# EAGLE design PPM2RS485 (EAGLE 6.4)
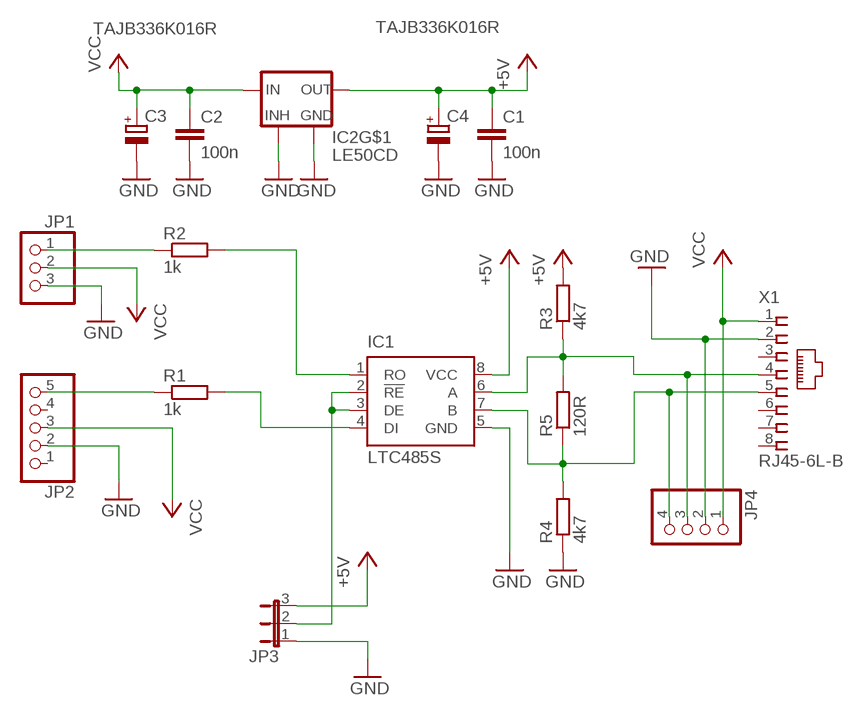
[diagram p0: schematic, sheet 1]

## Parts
C1  100n  C-EU_KOLIN  [M0805]
C2  100n  C-EU_KOLIN  [M0805]
C3  TAJB336K016R  CPOL-EUSMCB  [SMC_B]
C4  TAJB336K016R  CPOL-EUSMCB  [SMC_B]
IC1  LTC485S  [SOIC8]
IC2  LE50CD  LE33CD  [SO8]
JP1  PINHD-1X3  [1X03]
JP2  PINHD-1X5  [1X05]
JP3  JP2E  [JP2]
JP4  PINHD-1X4  [1X04]
R1  1k  R-EU_KOLINM0805  [M0805]
R2  1k  R-EU_KOLINM0805  [M0805]
R3  4k7  R-EU_KOLINM0805  [M0805]
R4  4k7  R-EU_KOLINM0805  [M0805]
R5  120R  R-EU_KOLINM0805  [M0805]
X1  RJ45-6L-B  [RJ45-NO-SHIELD]

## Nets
+5V: C1.1 C4.+ IC1.8(VCC) IC2.1(OUT) JP3.3 R3.2
GND: C1.2 C2.2 C3.- C4.- IC1.5(GND) IC2.5(INHIBIT) IC2.7(GND) JP1.3 JP2.2 JP3.1 JP4.2 R4.1 X1.2
N$1: IC1.7(B) JP4.4 R4.2 R5.1 X1.5
N$2: IC1.6(A) JP4.3 R3.1 R5.2 X1.4
N$3: IC1.2(!RE) IC1.3(DE) JP3.2
N$4: IC1.4(DI) R1.2
N$5: JP2.5 R1.1
N$6: IC1.1(RO) R2.2
N$7: JP1.1 R2.1
VCC: C2.1 C3.+ IC2.8(IN) JP1.2 JP2.3 JP4.1 X1.1
Unconnected: JP2.1 JP2.4 X1.3 X1.6 X1.7 X1.8

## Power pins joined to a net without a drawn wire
GND: IC2.2(GND) IC2.3(GND) IC2.6(GND)

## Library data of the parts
C1 C2 = PINHEAD_RC:C-EU_KOLIN: CAPACITOR, European symbol
C3 C4 = rcl:CPOL-EU: POLARIZED CAPACITOR, European symbol
IC1 = linear-technology:LTC485: Low Power RS485 Interface Transceiver Source: http://www.linear.com/pc/downloadDocument.do?navId=H0,C1,C1007,C1017,P2064,D1718; OC_FARNELL: unknown; OC_NEWARK: unknown
IC2 = libstabilizatory:LE33CD: VOLTAGE REGULATOR WITH INHIBIT
JP1 = pinhead-round:PINHD-1X3: PIN HEADER
JP2 = pinhead-round:PINHD-1X5: PIN HEADER
JP3 = jumper:JP2E: JUMPER
JP4 = pinhead-round:PINHD-1X4: PIN HEADER
R1-R5 = PINHEAD_RC:R-EU_KOLIN: RESISTOR, European symbol
X1 = con-tycoelectronics:RJ45: CORCOM Modular RJ Jacks No Shield Source: www.tycoelectronics.com .. ENG_DS_1654001_1099_RJ_L_0507.pdf; MPN: RJ45-6L-B; OC_FARNELL: unknown; OC_NEWARK: 16R6090

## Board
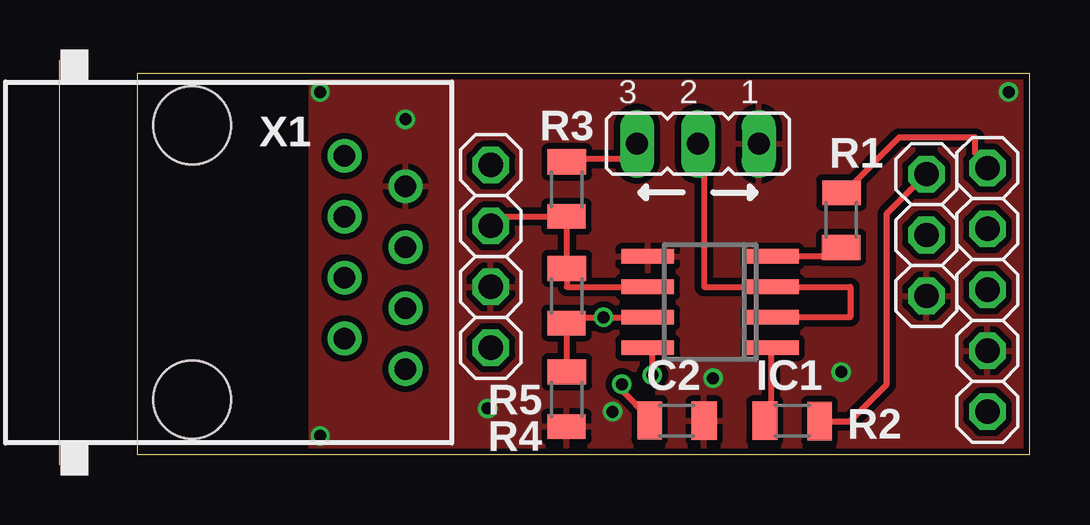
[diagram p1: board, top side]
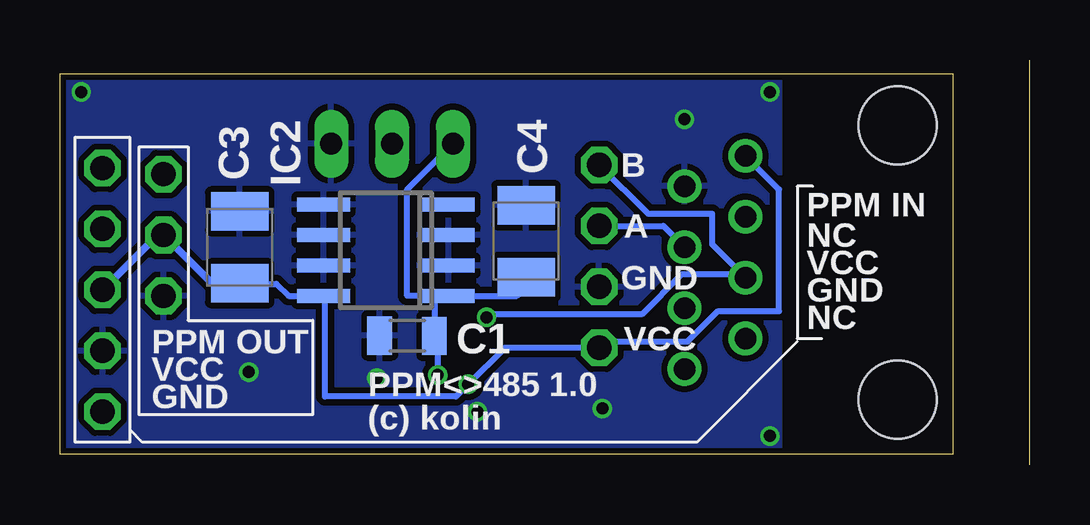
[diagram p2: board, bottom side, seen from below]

Size 40.44 x 16.89 mm. Coordinates in mm from the lower left corner, seen from the top.
Outline: 3.23,0.44 40.42,0.44 40.44,16.32 3.23,16.32 3.23,0.44
Copper layers (1*16): Top 0.035mm / dielectric 1.5mm / Bottom 0.035mm
Design rules "ITEADstudio_DRC": minimum track width 6mil, minimum drill 12mil, track to track 6mil, track to pad 6mil, pad to pad 6mil, via to via 6mil, smd to smd 0mil, copper to edge 10mil, drill to drill 10mil, minimum pad ring 10mil, minimum via ring 6mil, stop-mask expansion 2mil, vias tented up to drill 100mil, thermal gap 10mil

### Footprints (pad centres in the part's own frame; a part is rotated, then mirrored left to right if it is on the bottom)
M0805 = smd 1.021 x 1.6: 1 -1.131,0.017 | smd 1.046 x 1.6: 2 1.148,0
SMC_B = smd 1.6 x 2.4: + -1.5,0; - 1.5,0
SOIC8 = smd 0.6 x 2.2: 1 -1.905,-2.6; 2 -0.635,-2.6; 3 0.635,-2.6; 4 1.905,-2.6; 5 1.905,2.6; 6 0.635,2.6; 7 -0.635,2.6; 8 -1.905,2.6
SO8 = smd 0.6 x 2.2: 1 -1.905,-2.6; 2 -0.635,-2.6; 3 0.635,-2.6; 4 1.905,-2.6; 5 1.905,2.6; 6 0.635,2.6; 7 -0.635,2.6; 8 -1.905,2.6
1X03 = drill 1.016 octagon: 1 -2.54,0; 2 0,0; 3 2.54,0
1X05 = drill 1.016 octagon: 1 -5.08,0; 2 -2.54,0; 3 0,0; 4 2.54,0; 5 5.08,0
JP2 = drill 0.914 long: 1 -2.54,0; 2 0,0; 3 2.54,0
1X04 = drill 1.016 octagon: 1 -3.81,0; 2 -1.27,0; 3 1.27,0; 4 3.81,0
RJ45-NO-SHIELD = drill 0.9 pad 1.4: 1 -4.445,6.35; 2 -3.175,8.89; 3 -1.905,6.35; 4 -0.635,8.89; 5 0.635,6.35; 6 1.905,8.89; 7 3.175,6.35; 8 4.445,8.89 | hole 3.251: -5.715,0; 5.715,0

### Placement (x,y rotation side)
C1  25.96,5.4 180 bottom
C2  25.7,1.84 0 top
C3  32.94,9.08 90 bottom
C4  21.01,9.33 90 bottom
IC1  27.1,6.79 90 top
IC2  26.85,8.95 90 bottom
JP1  36.12,9.59 270 top
JP2  38.66,7.3 90 top
JP3  26.59,13.4 180 top
JP4  17.96,8.7 90 top
R1  32.56,10.22 270 top
R2  30.53,1.84 180 top
R3  21.13,11.49 90 top
R4  21.13,2.73 90 top
R5  21.13,7.05 90 top
X1  5.51,8.45 270 top

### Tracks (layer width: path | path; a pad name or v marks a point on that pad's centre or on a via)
+5V  (via drill 0.5)
  Top 0.254: JP3.3 24.05,12.76 21.13,12.76 R3.2 | v24.69,3.75 24.69,4.76 24.56,4.89 IC1.8
  Bottom 0.254: 24.82,7.05 24.82,5.4 C1.1 24.69,5.4 v24.69,3.75 | IC2.1 24.82,7.05 | IC2.1 21.39,7.05 20.62,7.81 C4.+ | JP3.3 25.96,11.49 25.96,7.05 24.82,7.05 | 24.31,7.05 IC2.1
GND  (via drill 0.5)
  other vias: 14.4,14.41 17.83,2.35 23.04,2.22 27.23,3.62 32.56,3.87 10.85,1.21 10.85,15.56 39.55,15.56
  pour Bottom (isolate 0.254): 10.46,0.44 40.44,0.44 40.44,16.32 10.46,16.32
  pour Top (isolate 0.254): 10.46,0.44 40.44,0.44 40.44,16.32 10.46,16.32
N$1  (via drill 0.5)
  Top 0.254: R4.2 21.13,5.91 R5.1 21.13,6.03 21.13,6.16 v22.66,6.16 IC1.7
  Bottom 0.254: JP4.4 15.93,10.48 13.26,10.48 13.26,9.21 X1.5 12.12,7.94 14.53,7.94 16.18,6.29 22.53,6.29 v22.66,6.16
N$2
  Top 0.254: IC1.6 21.13,7.43 R5.2 21.13,10.35 R3.1 21.01,10.35 17.96,10.35 JP4.3
  Bottom 0.254: X1.4 15.29,9.97 JP4.3
N$3
  Top 0.254: 29.77,6.16 IC1.2 32.94,6.16 32.94,7.43 IC1.3 26.85,7.43 26.85,12 26.59,12.26 JP3.2
N$4
  Top 0.254: R1.2 32.56,8.95 32.05,8.95 32.05,8.7 IC1.4
N$5
  Top 0.254: JP2.5 38.66,12.51 38.15,13.02 38.15,13.65 34.98,13.65 32.69,11.37 R1.1
N$6
  Top 0.254: R2.2 29.64,2.1 29.64,4.89 IC1.1
N$7
  Top 0.254: R2.1 32.93,1.82 34.47,3.37 34.47,10.48 JP1.1
VCC  (via drill 0.5)
  Top 0.254: v23.42,3.37 23.42,3.11 24.56,1.97 C2.1
  Bottom 0.254: C3.+ 32.69,7.56 31.42,7.56 30.91,7.05 IC2.8 29.39,7.05 29.39,2.86 23.93,2.86 v23.42,3.37 21.89,4.89 JP4.1 17.7,5.14 14.27,5.14 13,6.41 10.46,6.41 10.46,11.49 X1.1
  Bottom 0.305: C3.+ 34.11,7.58 JP1.2 36.37,9.59 JP2.3

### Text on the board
bPlace: B | PPM IN | NC | A | VCC | GND | GND | NC | VCC | PPM OUT | VCC | PPM<>485 1.0 | GND | (c) kolin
